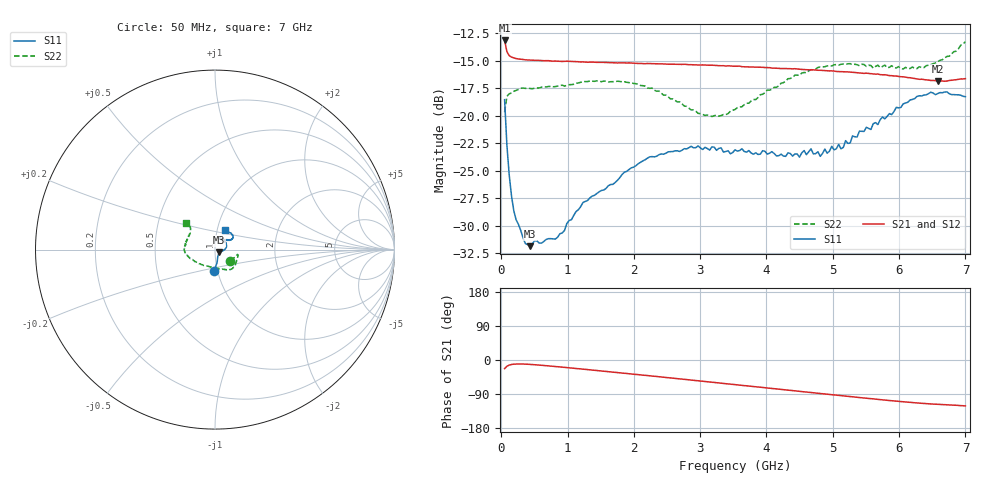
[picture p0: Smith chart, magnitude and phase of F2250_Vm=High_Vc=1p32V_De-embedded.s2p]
! Integrated Device Technology
! Corporate Headquarters
! 6024 Silver Creek Valley Road
! San Jose, CA 95138  USA
! Phone:  1-408-284-8200
! Toll Free:  1-800-223-1366
! Webpage:  http://www.idt.com/
! Timing and RF Division
! 515 Groton Road, Suite 102
! Westford, MA 01886-6024
! Device:  F2250
! Description: Voltage Variable RF Attenuator
! Frequency:  50.0 -  6000.00 MHz
! Package:  3x3 mm Thin QFN Plastic Package: 16 pin
! Ports:  2 RF, 3 DC
!  Pin  1  = GND
!  Pin  2  = NC
!  Pin  3  = RF1  = Port 1
!  Pin  4  = NC
!  Pin  5  = GND
!  Pin  6  = GND
!  Pin  7  = GND
!  Pin  8  = GND
!  Pin  9  = NC
!  Pin 10  = RF2  = Port 2
!  Pin 11  = NC
!  Pin 12  = GND
!  Pin 13  = GND
!  Pin 14  = VCNTRL
!  Pin 15  = VDD
!  Pin 16  = VMODE
! Vcntrl:  1.320 Volts
! Vmode:  +3.300 Volts
! Vdd:  +3.30  Volts
! Current:  1.332 mA
! Data:  The device was measured on a the F2250 evaluation board which has
!  individual transmission lines to the RF pins.  Data was collected
!  using a calibrated network analyzer.  The evaluation board was
!  de-embedded using a TRL calibration technique.
!  The reference plane is the edge of the package pin.
! Misc:  SN 10
!  Action Tracker AT0258
! Date Measured:  2014-11-26
! Date:  2015-10-15  MJV
! Note:
!  Integrated Device Technology supplies this data as a sample of measured
!  data at the package pin for this product.  Your particular data for this
!  product may vary.
!  Data was taken at 25 degrees C.
!  Integrated Device Technology reserves the right to change this data at anytime.
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# GHz S dB R 50
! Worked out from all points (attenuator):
!   201 points, 50 MHz to 7 GHz, reference 50 ohm
!   highest |S21| = -13.16 dB at 50 MHz (marker M1); lowest = -16.9 dB at 6.583 GHz (marker M2)
!   lowest |S11| = -31.9 dB at 432.2 MHz (marker M3), VSWR 1.05, Z = 52.1 - j1.52 ohm
!   |S11| at or under -10 dB: start of sweep to end of sweep
!   |S22| runs from -20.1 to -13.3 dB; largest |S21 - S12| = 0.0008
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0.05  -18.55 -92.6  -13.16 -22.8  -13.16 -22.8  -19.69 -36.1
0.08475  -22.72 -80.7  -14.19 -16.5  -14.18 -16.5  -18.25 -18.4
0.1195  -25.40 -75.0  -14.55 -13.4  -14.52 -13.4  -18.02 -13.7
0.189  -28.67 -62.2  -14.75 -11.0  -14.76 -11.0  -17.79 -12.2
0.36275  -31.64 -38.1  -14.93 -10.9  -14.92 -10.9  -17.52 -13.9
0.43225  -31.88 -34.9  -14.95 -11.6  -14.94 -11.6  -17.53 -15.2
0.84925  -31.06 -18.1  -15.05 -17.7  -15.03 -17.7  -17.32 -28.1
1.2315  -27.91 -12.7  -15.11 -24.1  -15.10 -24.2  -16.90 -37.7
1.857  -25.15 1.5  -15.20 -35.0  -15.20 -35.0  -16.92 -49.8
2.37825  -23.56 15.1  -15.29 -44.2  -15.30 -44.2  -17.76 -61.2
3.07325  -22.88 37.2  -15.40 -56.8  -15.38 -56.8  -19.99 -93.1
3.525  -23.11 52.7  -15.51 -65.0  -15.52 -65.0  -19.44 -123.6
4.498  -23.78 64.6  -15.79 -82.6  -15.79 -82.7  -16.33 -165.2
4.67175  -23.03 63.2  -15.85 -85.8  -15.84 -85.8  -15.82 -169.1
4.7065  -23.48 63.8  -15.84 -86.5  -15.85 -86.5  -15.84 -169.7
4.81075  -23.71 60.1  -15.88 -88.3  -15.88 -88.3  -15.56 -171.7
5.08875  -22.62 51.0  -15.99 -93.4  -15.98 -93.5  -15.40 -178.0
5.1235  -23.02 51.2  -15.99 -94.0  -15.99 -94.1  -15.34 -179.0
5.85325  -19.82 32.4  -16.36 -106.8  -16.36 -107.0  -15.61 163.6
6.27025  -18.25 33.8  -16.66 -113.4  -16.66 -113.4  -15.72 150.4
6.583  -17.99 41.0  -16.88 -116.9  -16.86 -117.0  -15.08 140.6
7  -18.28 63.7  -16.64 -121.1  -16.63 -121.3  -13.28 137.5
